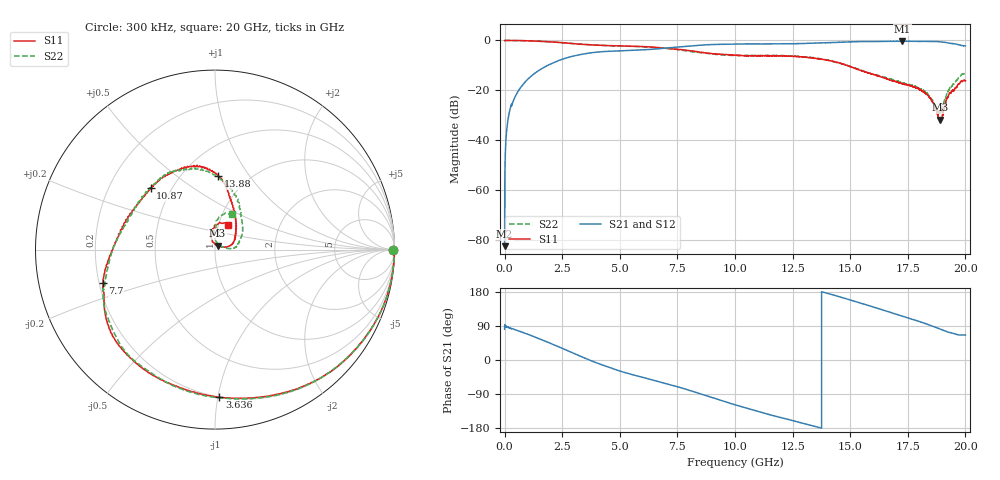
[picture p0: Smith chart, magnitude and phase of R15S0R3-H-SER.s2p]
!{R15S0R3}
!Johanson Technology Inc.
!www.johansontechnology.com
!Test Board Conditions:
!Substrate Type  RO4350B
!Substrate Thickness  20 mil
!Substrate Dk  3.66
!TL Type: GCPW
!TL Trace Width  34 mil
!TL Gap  10 mil
!Electrode orientation  Horizontal
!DUT TOPOLOGY	SERIES
!Mounting Pad LxW  26x52 mil
! Created Sat Feb  6 12:04:53 2021
# hz S ma R 50
! 2 Port Network Data from SP1.SP block
! freq  magS11  angS11  magS21  angS21  magS12  angS12  magS22  angS22
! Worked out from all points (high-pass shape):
!   20001 points, 300 kHz to 20 GHz, reference 50 ohm
!   highest |S21| = -0.28 dB at 17.27 GHz (marker M1); lowest = -82.3 dB at 300 kHz (marker M2)
!   |S21| within 3 dB of the highest: 6.734204 GHz to 6.737168 GHz (2.964 MHz wide, 0.044 % of centre); 6.737 GHz to end of sweep
!   lowest |S11| = -31.7 dB at 18.9 GHz (marker M3), VSWR 1.05, Z = 51.4 + j2.23 ohm
!   |S11| at or under -10 dB: 14.86 GHz to end of sweep
!   |S22| runs from -29.2 to 0.0 dB; largest |S21 - S12| = 0.016
!   S11 on the Smith chart (normalised r, x): 300 kHz: open; 3.636 GHz: 0.20, -1.01; 7.7 GHz: 0.21, -0.14; 10.87 GHz: 0.39, +0.35; 13.88 GHz: 0.73, +0.73; 20 GHz: 1.11, +0.31
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300000  0.9925 0.0  7.682e-05 81.2  0.0001309 125.0  0.9929 -0.1
1.023e8  0.9998 -2.4  0.01815 87.6  0.01824 87.5  0.9998 -2.3
1.423e8  0.9995 -3.1  0.02532 86.6  0.0254 86.6  0.9996 -3.2
2.733e8  0.9985 -6.4  0.04854 82.9  0.04881 83.0  0.9977 -6.4
5.303e8  0.996 -11.3  0.08691 78.4  0.08712 78.5  0.9955 -11.3
1.5633e9  0.9604 -35.2  0.264 54.6  0.265 54.5  0.9604 -35.1
3.3343e9  0.8402 -80.7  0.5269 8.8  0.5282 8.8  0.8412 -81.5
3.6363e9  0.8235 -88.3  0.5559 1.0  0.5564 1.0  0.8241 -89.6
5.0733e9  0.7759 -119.5  0.6212 -30.4  0.6221 -30.3  0.7684 -121.1
6.6673e9  0.7209 -147.0  0.6818 -56.7  0.6837 -56.5  0.7119 -145.8
7.7003e9  0.6524 -163.3  0.7496 -74.1  0.7534 -74.1  0.6378 -163.7
1.00003e10  0.5089 154.3  0.8469 -118.1  0.85 -118.1  0.5034 150.2
1.08693e10  0.4949 136.4  0.8518 -133.4  0.8532 -133.8  0.4989 136.5
1.33343e10  0.4483 93.8  0.8809 -173.2  0.8761 -173.3  0.4511 100.4
1.38833e10  0.412 87.4  0.8995 177.9  0.8887 178.0  0.4181 90.2
1.52423e10  0.2737 70.1  0.9419 154.1  0.9393 154.5  0.2777 60.5
1.66673e10  0.1668 44.6  0.9628 127.0  0.9585 127.6  0.1748 29.9
1.72673e10  0.1367 33.1  0.9678 115.6  0.9621 116.1  0.1417 18.5
1.82943e10  0.08602 14.5  0.9545 95.5  0.9585 95.6  0.08926 3.8
1.88993e10  0.02604 56.2  0.9411 81.8  0.9394 82.0  0.03558 55.0
1.92753e10  0.08179 102.4  0.8857 73.2  0.8916 73.6  0.09973 92.9
2e10  0.156 61.5  0.7792 66.0  0.7772 66.3  0.2198 63.4
